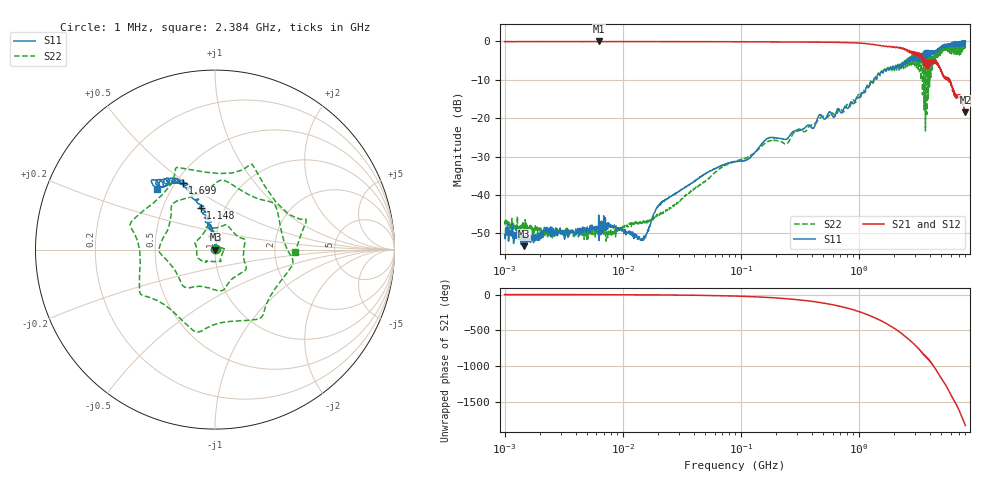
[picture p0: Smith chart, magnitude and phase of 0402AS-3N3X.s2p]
!s-Parameter Generated by FASTRON Sdn. Bhd.
!FASTRON P/N : 0402AS-3N3X
!Keysight Technologies: E5071C_MY46733604_B.14.02
!Date: Mon Dec 01 10:22:43 2025
!Version  :Rev00  Mon Dec 01 10:22:43 2025
!Data & Calibration Information:
!Freq  S11:SOLT2(ON)  S21:SOLT2(ON)  S12:SOLT2(ON)  S22:SOLT2(ON)
!PortZ  Port1:50+j0  Port2:50+j0
!When reading reference impedance value at option line is always used.
! Remarks : This data is being provided solely for informational purposes.
# Hz S dB R 50
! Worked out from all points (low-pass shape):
!   1601 points, 1 MHz to 8 GHz, reference 50 ohm
!   highest |S21| = 0.01 dB at 6.268 MHz (marker M1); lowest = -18.4 dB at 8 GHz (marker M2)
!   |S21| within 3 dB of the highest: start of sweep to 2.721 GHz; 2.735 GHz to 2.804 GHz (69.72 MHz wide, 2.52 % of centre)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
!   lowest |S11| = -53.3 dB at 1.468 MHz (marker M3), VSWR 1.00, Z = 50.2 + j0.032 ohm
!   |S11| at or under -10 dB: start of sweep to 1.334 GHz
!   |S22| runs from -52.0 to -0.4 dB; largest |S21 - S12| = 0.017
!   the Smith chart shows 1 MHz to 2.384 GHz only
!   S11 on the Smith chart (normalised r, x): 1 MHz: 1.01, +0.00; 1.148 GHz: 0.77, +0.38; 1.699 GHz: 0.54, +0.48; 2.384 GHz: 0.42, +0.36
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1000000  -50.40 31.1  -0.05 -0.3  -0.03 -0.3  -47.60 13.3
1468277  -53.30 8.5  -0.04 -0.4  -0.02 -0.4  -47.40 -2.8
4479405  -48.90 14.7  -0.04 -1.1  -0.02 -1.1  -49.80 20.3
6268472  -45.20 13.2  0.01 -1.2  -0.03 -1.2  -49.60 14.1
2.00676e7  -42.90 26.8  -0.05 -4.9  -0.04 -4.8  -45.20 59.3
8.994653e7  -31.30 90.8  -0.07 -21.7  -0.07 -21.7  -31.20 21.4
4.006501e8  -22.50 111.0  -0.17 -95.5  -0.15 -95.5  -21.70 -128.0
7.643634e8  -16.90 106.0  -0.29 178.0  -0.28 178.0  -17.50 74.8
1.14826e9  -12.20 109.0  -0.56 85.9  -0.56 85.9  -12.70 -117.0
1.699028e9  -7.71 116.0  -1.21 -43.0  -1.21 -43.0  -7.79 -24.4
1.7949e9  -7.46 118.0  -1.28 -65.2  -1.28 -65.2  -7.50 -70.0
2.018602e9  -6.72 127.0  -1.46 -119.0  -1.45 -119.0  -7.28 174.0
2.384191e9  -6.58 134.0  -1.71 154.0  -1.68 154.0  -7.01 -2.1
2.736325e9  -4.38 136.0  -2.99 72.1  -2.95 72.0  -3.90 -175.0
3.000426e9  -4.09 147.0  -3.35 8.7  -3.31 8.5  -5.06 40.4
3.284549e9  -4.07 154.0  -3.67 -61.1  -3.64 -61.4  -7.88 -108.0
3.791269e9  -2.47 158.0  -6.95 -164.0  -6.92 -164.0  -12.50 -10.4
4.240668e9  -2.72 170.0  -5.67 87.7  -5.68 87.2  -2.92 -165.0
4.57657e9  -2.38 171.0  -5.38 10.0  -5.41 9.6  -4.48 18.8
4.968456e9  -1.33 -176.0  -7.55 -85.0  -7.58 -85.3  -2.76 176.0
5.360342e9  -0.71 -160.0  -9.61 -169.0  -9.65 -169.0  -1.96 -5.3
8e9  0.06 -78.9  -18.40 -35.0  -18.40 -35.2  -1.79 173.0
